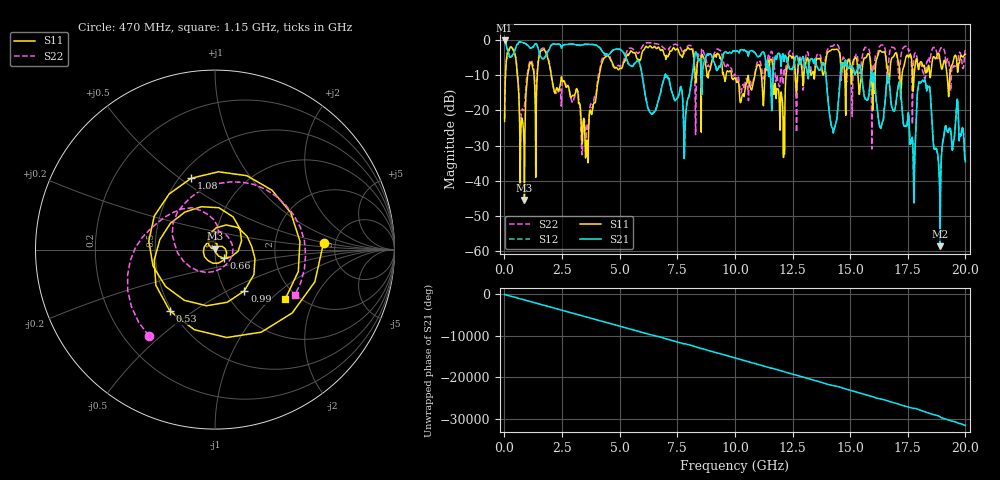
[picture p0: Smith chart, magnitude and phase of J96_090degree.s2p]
!Keysight Technologies,N5222A,MY51421036,A.10.65.16
!Date: Friday, March 31, 2023 14:23:08
!Correction: S11(Full 2 Port(1,2))
!S21(Full 2 Port(1,2))
!S12(Full 2 Port(1,2))
!S22(Full 2 Port(1,2))
!S2P File: Measurements: S11, S21, S12, S22:
# Hz S  dB  R 50
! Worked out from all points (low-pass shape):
!   2000 points, 10 MHz to 20 GHz, reference 50 ohm
!   highest |S21| = -0.21 dB at 10 MHz (marker M1); lowest = -58.5 dB at 18.9 GHz (marker M2)
!   |S21| within 3 dB of the highest: 438.9 MHz to 1.497 GHz (1.058 GHz wide, 109 % of centre); 1.898 GHz to 4.237 GHz (2.34 GHz wide, 76.3 % of centre)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
!   lowest |S11| = -45.5 dB at 870 MHz (marker M3), VSWR 1.01, Z = 50 + j0.534 ohm
!   |S11| at or under -10 dB: 2.027 GHz to 4.117 GHz (2.09 GHz wide, 68 % of centre); 9.85 GHz to 10.87 GHz (1.017 GHz wide, 9.82 % of centre); 11.66 GHz to 12.22 GHz (561 MHz wide, 4.7 % of centre)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
!   |S22| runs from -32.6 to -0.8 dB; largest |S21 - S12| = 0.012
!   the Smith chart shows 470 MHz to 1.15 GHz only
!   S11 on the Smith chart (normalised r, x): 470 MHz: 4.01, +0.47; 530 MHz: 0.49, -0.40; 660 MHz: 1.10, -0.11; 990 MHz: 1.22, -0.61; 1.08 GHz: 0.57, +0.55; 1.15 GHz: 1.72, -1.24
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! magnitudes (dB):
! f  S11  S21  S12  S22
! 10 MHz  -23.2  -0.2  -0.3  -22.4
! 470 MHz  -4.4  -2.7  -2.7  -4.4
! 530 MHz  -7.5  -1.5  -1.5  -7.0
! 660 MHz  -23.3  -0.6  -0.6  -21.9
! 870 MHz  -45.5  -1.0  -1.0  -19.1
! 990 MHz  -11.0  -1.4  -1.4  -9.9
! 1.08 GHz  -7.6  -2.1  -2.1  -6.6
! 1.15 GHz  -6.4  -2.4  -2.4  -5.8
! 3.35 GHz  -26.9  -1.5  -1.4  -31.2
! 4.34 GHz  -5.1  -4.0  -4.0  -4.4
! 6.68 GHz  -2.1  -17.2  -17.2  -1.3
! 10.01 GHz  -10.8  -3.3  -3.3  -9.8
! 13.34 GHz  -9.6  -5.4  -5.4  -9.5
! 14.26 GHz  -2.8  -26.1  -26.1  -1.8
! 14.71 GHz  -6.8  -7.4  -7.4  -4.9
! 16.33 GHz  -3.2  -25.2  -25.1  -1.5
! 16.67 GHz  -11.2  -10.8  -10.7  -6.2
! 17.72 GHz  -13.5  -30.0  -29.8  -12.8
! 18.35 GHz  -9.1  -13.2  -13.1  -6.2
! 18.9 GHz  -5.7  -58.5  -54.2  -2.7
! 19.61 GHz  -5.2  -19.8  -19.8  -7.4
! 20 GHz  -4.1  -34.5  -34.9  -2.9
